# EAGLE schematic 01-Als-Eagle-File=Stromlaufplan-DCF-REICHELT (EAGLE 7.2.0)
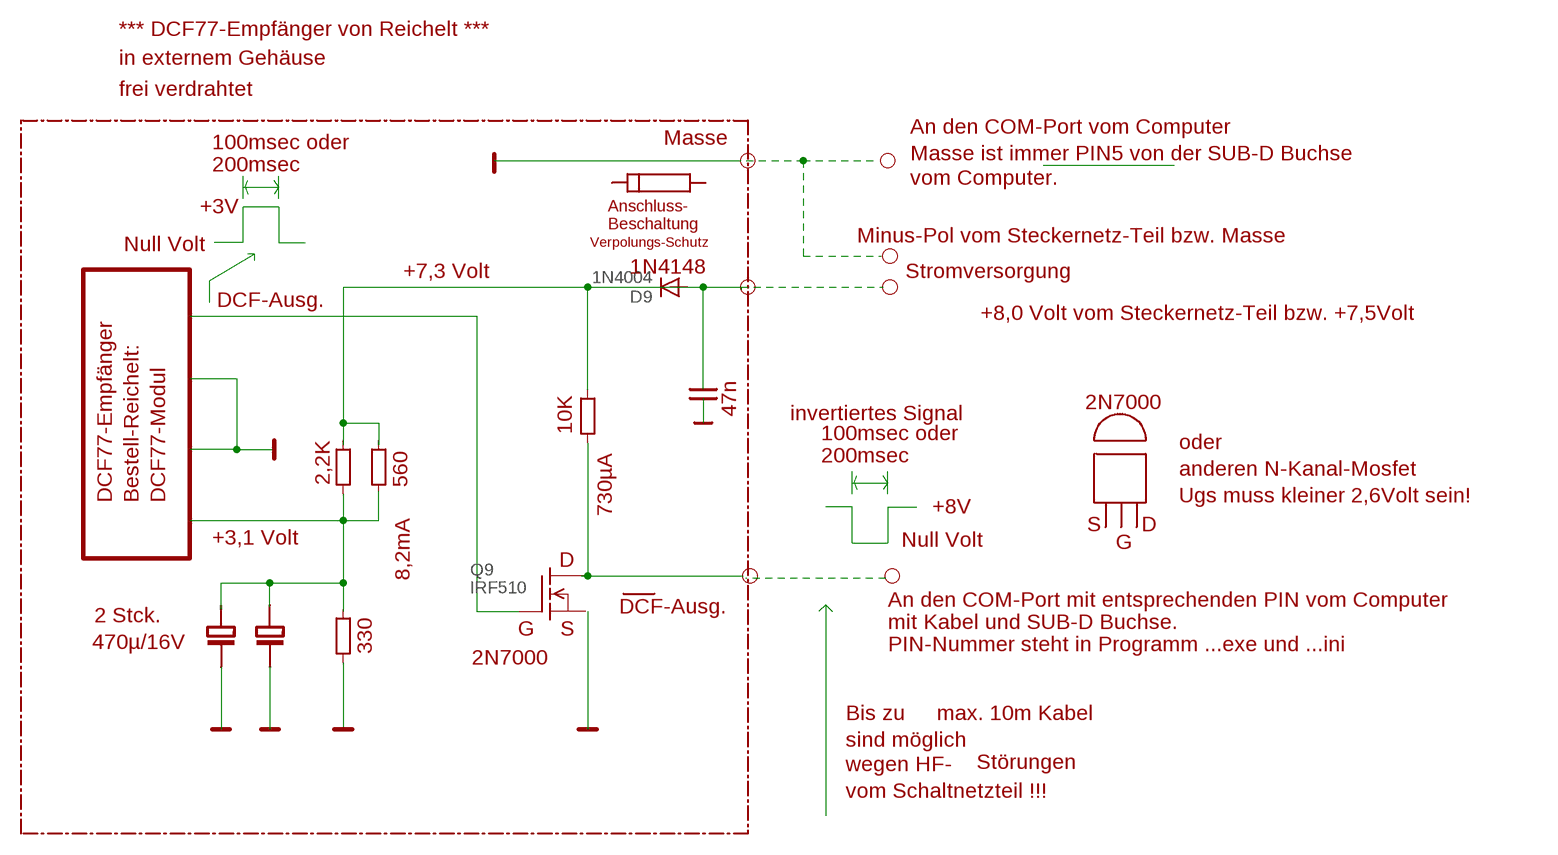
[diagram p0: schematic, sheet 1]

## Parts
D9  1N4004  [DO41-10]
Q9  IRF510  [TO220]

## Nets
N$197: Q9.2(D)
N$210: Q9.1(G)
N$217: D9.A D9.C
Unconnected: Q9.3(S)

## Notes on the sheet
- *** DCF77-Empfänger von Reichelt ***
- in externem Gehäuse
- frei verdrahtet
- An den COM-Port vom Computer
- 100msec oder | Masse
- Masse ist immer PIN5 von der SUB-D Buchse
- 200msec
- vom Computer.
- +3V
- Anschluss-
- Beschaltung
- Null Volt
- Minus-Pol vom Steckernetz-Teil bzw. Masse
- Verpolungs-Schutz
- +7,3 Volt | 1N4148 | Stromversorgung
- DCF-Ausg. | +8,0 Volt vom Steckernetz-Teil bzw. +7,5Volt
- 47n
- 2N7000
- invertiertes Signal
- 10K
- 100msec oder
- oder
- 200msec
- anderen N-Kanal-Mosfet
- 2,2K | 560
- DCF77-Empfänger | Bestell-Reichelt: | DCF77-Modul | Ugs muss kleiner 2,6Volt sein!
- 730µA | +8V
- S | D
- +3,1 Volt | Null Volt | G
- D
- 8,2mA
- An den COM-Port mit entsprechenden PIN vom Computer
- DCF-Ausg.
- 2 Stck.
- mit Kabel und SUB-D Buchse.
- G | S
- 470µ/16V | 330 | PIN-Nummer steht in Programm ...exe und ...ini
- 2N7000
- Bis zu | max. 10m Kabel
- sind möglich
- wegen HF- | Störungen
- vom Schaltnetzteil !!!

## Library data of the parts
D9 = diode:1N4004: DIODE
Q9 = transistor-fet:IRF510: N-Channel Enhancement MOSFET (HEXFET); 100V; 5,6A; 0,54Ohm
